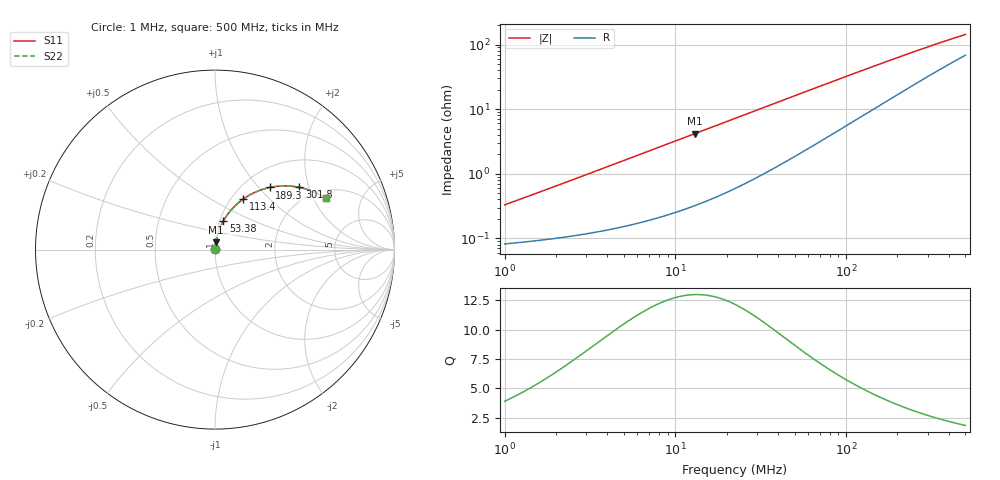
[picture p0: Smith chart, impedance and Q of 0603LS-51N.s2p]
# MHz S MA R 50
!Freq  MagS11  AngS11  MagS21  AngS21  MagS12  AngS12  MagS22  AngS22
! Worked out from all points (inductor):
!   801 points, 1 MHz to 500 MHz, reference 50 ohm
!   read as one part in series: L = 50.9 nH near 1.032 MHz
!   highest Q = 13 at 12.98 MHz (marker M1), where L = 51 nH
!   S11 on the Smith chart (normalised r, x): 1 MHz: 1.00, +0.01; 53.38 MHz: 1.04, +0.34; 113.4 MHz: 1.13, +0.71; 189.3 MHz: 1.31, +1.15; 301.8 MHz: 1.64, +1.73; 500 MHz: 2.36, +2.52
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1  0.003299 75.4  0.9992 -0.2  0.9992 -0.2  0.003299 75.4
1.031561  0.003398 75.7  0.9992 -0.2  0.9992 -0.2  0.003398 75.7
1.302286  0.004252 77.9  0.9991 -0.2  0.9991 -0.2  0.004252 77.9
2.831897  0.009117 82.3  0.9988 -0.5  0.9988 -0.5  0.009117 82.3
7.957584  0.02548 83.9  0.9976 -1.5  0.9976 -1.5  0.02548 83.9
12.98151  0.04153 83.2  0.996 -2.4  0.996 -2.4  0.04153 83.2
22.53506  0.07192 81.2  0.9915 -4.1  0.9915 -4.1  0.07192 81.2
35.08814  0.1112 78.1  0.9831 -6.4  0.9831 -6.4  0.1112 78.1
53.37536  0.1663 73.7  0.9665 -9.5  0.9665 -9.5  0.1663 73.7
63.32315  0.195 71.3  0.9557 -11.1  0.9557 -11.1  0.195 71.3
73.96678  0.2244 68.9  0.9429 -12.8  0.9429 -12.8  0.2244 68.9
85.73088  0.2555 66.4  0.9277 -14.6  0.9277 -14.6  0.2555 66.4
98.59709  0.2876 63.7  0.91 -16.5  0.91 -16.5  0.2876 63.7
113.3942  0.3222 60.8  0.8887 -18.5  0.8887 -18.5  0.3222 60.8
140.9467  0.3799 55.9  0.8476 -21.8  0.8476 -21.8  0.3799 55.9
177.937  0.4447 50.2  0.7924 -25.5  0.7924 -25.5  0.4447 50.2
189.3459  0.462 48.6  0.7758 -26.5  0.7758 -26.5  0.462 48.6
239.0382  0.5255 42.5  0.7078 -30.1  0.7078 -30.1  0.5255 42.5
301.7718  0.5837 36.5  0.6338 -33.2  0.6338 -33.2  0.5837 36.5
399.1465  0.6429 29.7  0.544 -35.8  0.544 -35.8  0.6429 29.7
466.2368  0.6703 26.2  0.4965 -36.6  0.4965 -36.6  0.6703 26.2
500  0.6813 24.7  0.4761 -36.8  0.4761 -36.8  0.6813 24.7
